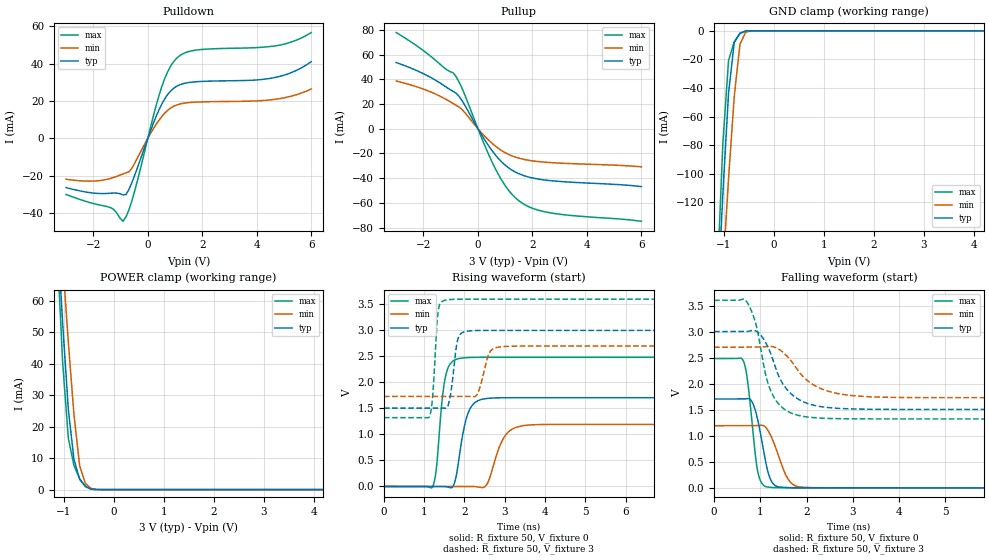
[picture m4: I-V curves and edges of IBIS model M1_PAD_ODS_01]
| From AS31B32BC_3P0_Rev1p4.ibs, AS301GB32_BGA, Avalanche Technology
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[Model] M1_PAD_ODS_01
Model_type I/O
Enable   Active-High
Vinl  =  0.8
Vinh  =  2.2
Vmeas =  1.5
Cref  =  30e-12
| Capacitance  typ   min   max
C_comp   1.536816e-12   1.424706e-12   1.652746e-12
| Variables   typ   min   max
[GND Clamp Reference]   0   0   0
[POWER Clamp Reference]   3   2.7   3.6
[Pulldown Reference]   0   0   0
[Pullup Reference]   3   2.7   3.6
[Temperature Range]   25   125   -40
[Voltage Range]   3   2.7   3.6
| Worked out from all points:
|   slope of the pulldown table from 0 to 0.45 V, typ, clamps not added: 27.4 ohm
|   slope of the pullup table from 0 to 0.45 V, typ, clamps not added: 28.8 ohm
|   GND clamp passes 1 mA (typ) near -0.63 V on its own axis
|   POWER clamp passes 1 mA (typ) near -0.57 V on its own axis
|   falling waveform, R_fixture 50, V_fixture 0: 20-80 % time 225ps typ, 305ps min, 176ps max; typ from 1.71 V to 0 V
|   falling waveform, R_fixture 50, V_fixture 3: 20-80 % time 499ps typ, 660ps min, 366ps max; typ from 3 V to 1.51 V
|   rising waveform, R_fixture 50, V_fixture 0: 20-80 % time 243ps typ, 335ps min, 176ps max; typ from 0 V to 1.71 V
|   rising waveform, R_fixture 50, V_fixture 3: 20-80 % time 138ps typ, 193ps min, 104ps max; typ from 1.51 V to 3 V
[GND Clamp]
| Voltage   I(typ)   I(min)   I(max)
-3V       -1.712A    -1.49A     -2.05A
-1.138V   -196mA     -238.3mA   -175.4mA
-1.024V   -114.1mA   -169mA     -78.8mA
-910.3mV  -43.65mA   -103.4mA   -20.77mA
-796.6mV  -8.267mA   -46.07mA   -7.668mA
-682.8mV  -1.833mA   -9.55mA    -1.767mA
-569mV    -178.4uA   -969.7uA   -71.94uA
-455.2mV  -3.831uA   -72.48uA   -403.8nA
6V        0A         0A         0A
[POWER Clamp]
| Voltage   I(typ)   I(min)   I(max)
-3V       673.8mA    591mA      808.5mA
-1.138V   84.79mA    99.96mA    78.44mA
-1.024V   53.08mA    72.89mA    40.56mA
-910.3mV  25.62mA    46.98mA    16.4mA
-796.6mV  9.531mA    23.75mA    7.632mA
-682.8mV  3.235mA    7.564mA    3.468mA
-569mV    995.3uA    1.941mA    1.029mA
-455.2mV  154.7uA    390.4uA    112.5uA
-227.6mV  35.58nA    2.313uA    2.593nA
6V        0A         0A         0A
[Pulldown]
| Voltage   I(typ)   I(min)   I(max)
-3V       -26.36mA   -21.88mA   -30.04mA
-1.366V   -29.37mA   -21.44mA   -37.07mA
-910.3mV  -30.26mA   -19.02mA   -44.4mA
-796.6mV  -30.03mA   -18.45mA   -41.9mA
-569mV    -23.1mA    -15.63mA   -32.68mA
206.9mV   8.128mA    5.203mA    12.16mA
517.2mV   18.44mA    11.77mA    27.81mA
724.1mV   23.38mA    14.96mA    35.49mA
1.034V    27.67mA    17.73mA    42.54mA
1.759V    30.28mA    19.41mA    47.23mA
4.614V    32.42mA    20.8mA     49.33mA
6V        41.08mA    26.43mA    56.64mA
[Pullup]
| Voltage   I(typ)   I(min)   I(max)
-3V       53.53mA    38.58mA    77.79mA
-1.821V   42.49mA    30.53mA    60.12mA
-910.3mV  30.2mA     20.33mA    45.32mA
-796.6mV  28.64mA    18.81mA    41.96mA
-569mV    22.26mA    15.27mA    32mA
206.9mV   -7.586mA   -5.1mA     -11.3mA
620.7mV   -20.68mA   -13.72mA   -31.55mA
1.034V    -30.14mA   -19.8mA    -47.15mA
1.552V    -36.89mA   -24.12mA   -59.12mA
2.069V    -40.18mA   -26.23mA   -64.93mA
2.69V     -42.09mA   -27.45mA   -68.2mA
6V        -46.88mA   -30.86mA   -74.94mA
[Ramp]
dV/dt_r   1.02353/0.242588n  0.715782/0.335331n  1.48949/0.176355n
dV/dt_f   0.896545/0.498993n  0.581576/0.659988n  1.3662/0.365774n
R_load = 50
[Falling Waveform]
R_fixture = 50
V_fixture = 0
V_fixture_min = 0
V_fixture_max = 0
| Time   V(typ)   V(min)   V(max)
0s        1.706V     1.193V     2.482V
635.9ps   1.706V     1.193V     2.431V
733.7ps   1.715V     1.193V     1.989V
940.8ps   1.318V     1.196V     323.6mV
1.028ns   923.9mV    1.201V     93.61mV
1.162ns   313.3mV    1.107V     14.87mV
1.307ns   52.56mV    830.3mV    5.36mV
1.596ns   5.342mV    172.7mV    1.351mV
1.955ns   1.195mV    9.401mV    393uV
21.88ns   -243.5nV   -824.1nV   -402.1nV
[Falling Waveform]
R_fixture = 50
V_fixture = 3
V_fixture_min = 2.7
V_fixture_max = 3.6
| Time   V(typ)   V(min)   V(max)
0s        3V         2.7V       3.6V
680.8ps   3.001V     2.7V       3.601V
875.3ps   3.017V     2.701V     3.232V
1.005ns   2.936V     2.702V     2.692V
1.133ns   2.761V     2.714V     2.105V
1.288ns   2.409V     2.705V     1.747V
1.582ns   1.881V     2.525V     1.473V
2.081ns   1.604V     2.016V     1.353V
3.936ns   1.506V     1.736V     1.323V
21.88ns   1.506V     1.731V     1.323V
[Rising Waveform]
R_fixture = 50
V_fixture = 0
V_fixture_min = 0
V_fixture_max = 0
| Time   V(typ)   V(min)   V(max)
0s        4.672nV    63.6nV     -79.24nV
1.21ns    809.7uV    36.26uV    -2.765mV
1.529ns   -1.101mV   45.8uV     2.116V
1.75ns    64.19mV    52.42uV    2.428V
1.918ns   823.3mV    57.42uV    2.467V
2.263ns   1.615V     -2.432mV   2.481V
2.568ns   1.693V     56.43mV    2.482V
3.05ns    1.705V     1.015V     2.482V
3.576ns   1.706V     1.179V     2.482V
21.88ns   1.706V     1.193V     2.482V
[Rising Waveform]
R_fixture = 50
V_fixture = 3
V_fixture_min = 2.7
V_fixture_max = 3.6
| Time   V(typ)   V(min)   V(max)
0s        1.506V     1.731V     1.323V
1.129ns   1.507V     1.731V     1.34V
1.203ns   1.507V     1.731V     1.679V
1.346ns   1.507V     1.731V     3.368V
1.581ns   1.536V     1.732V     3.588V
1.832ns   2.825V     1.732V     3.598V
2.138ns   2.991V     1.731V     3.599V
2.643ns   2.999V     2.598V     3.599V
2.983ns   2.999V     2.689V     3.599V
21.88ns   3V         2.7V       3.6V
